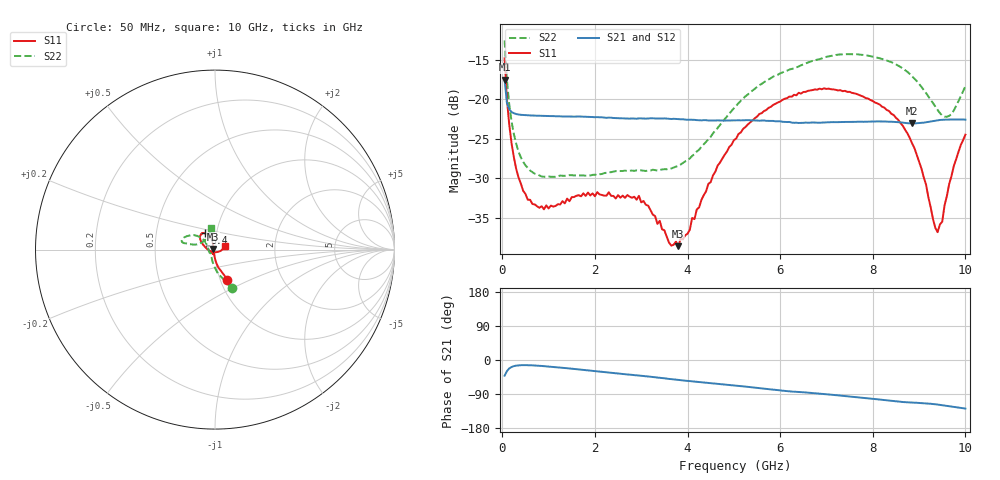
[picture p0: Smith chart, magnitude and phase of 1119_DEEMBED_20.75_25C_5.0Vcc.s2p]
!Hittite Microwave Corp.
!Digital Attenuator/PhaseShifter Rev 1.4.0
!Filename: C:\DATA\DATA\1119_DEEMBED_20.75_25C_5.0Vcc.s2p
!VNA ID: Agilent Technologies,N5224A,MY51441122,A.10.45.03
!Device type:
!2 Port Calibration.
!Temp(C): 25
!Lot Number:
!Serial Number:
!Operator:
!Misc:
!Attenuator:  20.750
# GHZ S DB R 50.0
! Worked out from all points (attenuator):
!   200 points, 50 MHz to 10 GHz, reference 50 ohm
!   highest |S21| = -17.54 dB at 50 MHz (marker M1); lowest = -23.1 dB at 8.85 GHz (marker M2)
!   lowest |S11| = -38.6 dB at 3.8 GHz (marker M3), VSWR 1.02, Z = 48.9 + j0.281 ohm
!   |S11| at or under -10 dB: start of sweep to end of sweep
!   |S22| runs from -29.8 to -12.6 dB; largest |S21 - S12| = 0.00026
!   S11 on the Smith chart (normalised r, x): 50 MHz: 1.08, -0.37; 6.4 GHz: 0.88, +0.17; 10 GHz: 1.12, +0.04
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0.05  -14.85 -67.4  -17.54 -41.5  -17.55 -41.5  -12.59 -66.4
0.1  -20.06 -79.9  -20.48 -29.4  -20.47 -29.4  -17.55 -83.3
0.2  -25.60 -89.6  -21.63 -18.5  -21.63 -18.4  -22.83 -100.0
0.35  -29.89 -96.7  -21.95 -14.2  -21.95 -14.1  -26.63 -114.0
0.55  -32.72 -104.7  -22.05 -13.7  -22.05 -13.6  -28.71 -125.6
0.9  -33.93 -112.6  -22.12 -16.3  -22.13 -16.2  -29.81 -134.8
1.75  -31.91 -124.3  -22.23 -26.2  -22.22 -26.2  -29.65 -139.5
2.95  -32.23 -124.8  -22.44 -40.9  -22.45 -41.0  -29.03 -158.5
3.4  -35.39 -145.4  -22.46 -46.9  -22.46 -47.0  -28.96 -171.9
3.6  -38.14 -165.8  -22.49 -49.9  -22.50 -50.0  -28.83 -179.4
3.8  -38.59 165.8  -22.53 -52.5  -22.53 -52.6  -28.44 172.3
5.05  -24.99 109.6  -22.69 -67.5  -22.70 -67.6  -20.84 139.6
5.55  -21.89 113.5  -22.73 -74.2  -22.74 -74.3  -18.25 141.9
6.4  -19.20 121.8  -23.02 -84.3  -23.03 -84.4  -15.88 150.7
6.7  -18.86 126.3  -22.96 -87.3  -22.97 -87.3  -15.17 154.6
7.5  -19.08 139.1  -22.88 -96.4  -22.89 -96.4  -14.32 163.9
8.35  -21.50 152.3  -22.86 -107.1  -22.86 -107.0  -15.22 168.0
8.85  -25.61 167.8  -23.08 -112.3  -23.08 -112.3  -17.12 167.6
9.400001  -36.82 -94.6  -22.69 -117.5  -22.70 -117.6  -21.37 153.5
9.5  -35.50 -51.6  -22.62 -119.3  -22.63 -119.4  -22.08 144.1
9.7  -29.72 -12.1  -22.58 -122.8  -22.60 -122.8  -21.88 121.0
10  -24.50 19.4  -22.60 -128.2  -22.61 -128.1  -18.34 99.5
